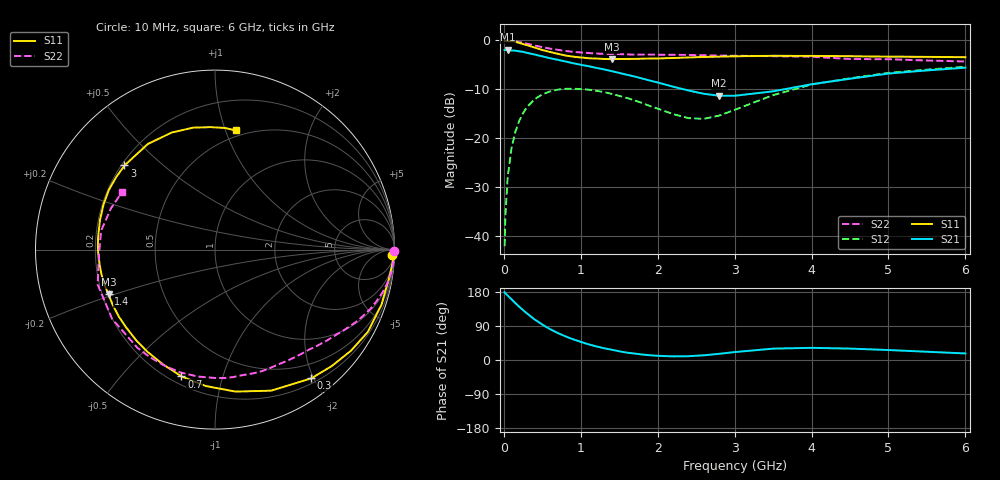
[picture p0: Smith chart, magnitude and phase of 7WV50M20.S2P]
! Infineon Technologies  Discrete & RF Semiconductors
! BFS17W
! Si NPN RF Bipolar Junction Transistor in SOT323
! VCE = 0.5 V  IC = 0.2 mA
! Common Emitter S-Parameters:  August  1999
# GHz  S  MA  R  50
!  f  S11  S21  S12  S22
! GHz  MAG  ANG  MAG  ANG  MAG  ANG  MAG  ANG
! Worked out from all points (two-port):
!   36 points, 10 MHz to 6 GHz, reference 50 ohm
!   highest |S21| = -1.91 dB at 50 MHz (marker M1); lowest = -11.3 dB at 2.8 GHz (marker M2)
!   |S21| within 3 dB of the highest: start of sweep to 978.4 MHz
!   lowest |S11| = -3.8 dB at 1.4 GHz (marker M3), VSWR 4.61, Z = 11.3 - j9.59 ohm
!   |S11| at or under -10 dB: nowhere
!   |S22| runs from -4.3 to 0.0 dB; largest |S21 - S12| = 0.8
!   S11 on the Smith chart (normalised r, x): 10 MHz: 22, -59; 300 MHz: 0.27, -1.97; 700 MHz: 0.24, -0.74; 1.4 GHz: 0.23, -0.19; 3 GHz: 0.21, +0.38; 6 GHz: 0.45, +1.09
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0.01  0.9892 -1.7  0.798 178.9  0.0079 88.5  0.9999 -0.3
0.02  0.9934 -3.9  0.798 176.1  0.016 86.2  0.9984 -1.5
0.05  0.9825 -9.4  0.803 169.9  0.04 84.3  0.9965 -3.8
0.1  0.9772 -18.3  0.789 160.2  0.0797 77.5  0.9901 -7.6
0.15  0.9671 -28.3  0.787 150.1  0.1166 70.6  0.9775 -11.2
0.3  0.8957 -53.2  0.747 123.0  0.2081 54.3  0.9275 -20.8
0.4  0.8459 -68.3  0.718 107.0  0.2511 44.6  0.8895 -26.4
0.5  0.7992 -81.8  0.688 93.6  0.2809 36.3  0.8544 -31.0
0.7  0.7307 -104.8  0.634 71.3  0.3145 23.4  0.8022 -39.3
0.9  0.6831 -123.1  0.585 54.6  0.3209 13.4  0.7645 -46.9
1.1  0.6583 -138.5  0.546 41.4  0.3144 5.7  0.7442 -54.4
1.4  0.6436 -157.2  0.486 27.0  0.2847 -2.5  0.7276 -65.9
1.8  0.6508 -177.8  0.408 14.4  0.229 -6.7  0.7173 -82.0
2.2  0.6615 165.6  0.337 9.5  0.1768 0.6  0.7138 -97.8
2.6  0.6783 150.6  0.285 12.4  0.1582 21.1  0.705 -113.7
2.8  0.6829 143.6  0.272 16.3  0.1706 31.4  0.7005 -121.3
3  0.6884 137.1  0.272 20.9  0.1953 38.9  0.6973 -128.4
3.5  0.6974 122.4  0.302 30.0  0.2761 44.7  0.691 -146.1
4  0.6953 110.3  0.357 32.1  0.3547 41.2  0.682 -163.4
4.5  0.6903 100.1  0.406 30.1  0.411 35.5  0.6465 -178.2
5.5  0.6799 85.4  0.494 21.8  0.5033 24.6  0.6236 158.4
6  0.6739 80.0  0.527 17.3  0.5386 19.4  0.6094 148.3
